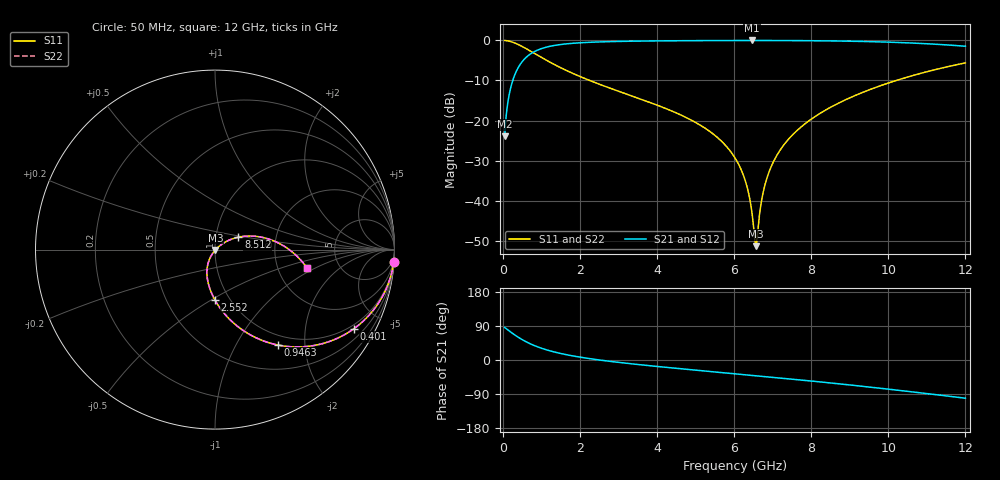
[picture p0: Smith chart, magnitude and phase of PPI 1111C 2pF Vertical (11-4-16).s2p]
# GHz S MA R 50
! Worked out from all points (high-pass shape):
!   1601 points, 50 MHz to 12 GHz, reference 50 ohm
!   highest |S21| = -0.03 dB at 6.466 GHz (marker M1); lowest = -23.9 dB at 50 MHz (marker M2)
!   |S21| within 3 dB of the highest: 778.9 MHz to end of sweep
!   lowest |S11| = -51.3 dB at 6.57 GHz (marker M3), VSWR 1.01, Z = 50.2 - j0.163 ohm
!   |S11| at or under -10 dB: 2.257 GHz to 10.21 GHz (7.948 GHz wide, 128 % of centre)
!   |S22| runs from -51.3 to 0.0 dB; largest |S21 - S12| = 0
!   S11 on the Smith chart (normalised r, x): 50 MHz: 1, -29; 401 MHz: 0.84, -3.58; 946.2 MHz: 0.84, -1.50; 2.552 GHz: 0.85, -0.52; 8.512 GHz: 1.28, +0.18; 12 GHz: 2.93, -0.84
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0.05  0.998 -4.0  0.06368 86.0  0.06368 86.0  0.998 -4.0
0.199375  0.9691 -15.6  0.2466 74.4  0.2466 74.4  0.9691 -15.6
0.4010313  0.8898 -29.8  0.4558 60.2  0.4558 60.2  0.8898 -29.8
0.6400313  0.7734 -43.5  0.6332 46.4  0.6332 46.4  0.7734 -43.5
0.94625  0.6354 -56.7  0.7713 33.2  0.7713 33.2  0.6354 -56.7
1.416781  0.4788 -70.6  0.8767 19.2  0.8767 19.2  0.4788 -70.6
2.044156  0.3481 -82.9  0.936 6.9  0.936 6.9  0.3481 -82.9
2.552031  0.2789 -90.3  0.9587 -0.6  0.9587 -0.6  0.2789 -90.3
4.038312  0.1538 -106.7  0.986 -17.4  0.986 -17.4  0.1538 -106.7
5.300531  0.0774 -117.9  0.9944 -29.6  0.9944 -29.6  0.0774 -117.9
6.025  0.03424 -122.1  0.9966 -36.3  0.9966 -36.3  0.03424 -122.1
6.301344  0.01719 -120.2  0.9969 -38.9  0.9969 -38.9  0.01719 -120.2
6.465656  0.007064 -108.3  0.997 -40.5  0.997 -40.5  0.007064 -108.3
6.525406  0.003804 -86.0  0.9969 -41.1  0.9969 -41.1  0.003804 -86.0
6.570219  0.002719 -36.8  0.9969 -41.5  0.9969 -41.5  0.002719 -36.8
6.771875  0.01382 35.0  0.9968 -43.4  0.9968 -43.4  0.01382 35.0
7.003406  0.02943 38.8  0.9963 -45.6  0.9963 -45.6  0.02943 38.8
7.414187  0.05872 37.4  0.9948 -49.6  0.9948 -49.6  0.05872 37.4
8.019156  0.1056 32.6  0.9907 -55.6  0.9907 -55.6  0.1056 32.6
8.512094  0.1474 27.9  0.9851 -60.7  0.9851 -60.7  0.1474 27.9
10.01331  0.2953 12.1  0.9506 -77.0  0.9506 -77.0  0.2953 12.1
12  0.5239 -11.4  0.8457 -100.8  0.8457 -100.8  0.5239 -11.4
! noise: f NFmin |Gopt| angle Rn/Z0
0.05  0.0006781  0.9446  2.351  0.002737
1.372  0.004053  0.6979  11.22  0.002598
2.701  0.006407  0.6399  19.34  0.003269
4.031  0.008532  0.6125  27.3  0.003873
5.36  0.0106  0.6016  34.91  0.004492
6.682  0.0127  0.6021  42.05  0.005176
8.012  0.01494  0.6113  48.76  0.005984
9.341  0.01737  0.6276  55.02  0.006973
10.67  0.0201  0.6495  60.88  0.008221
12  0.02323  0.6759  66.39  0.009839
